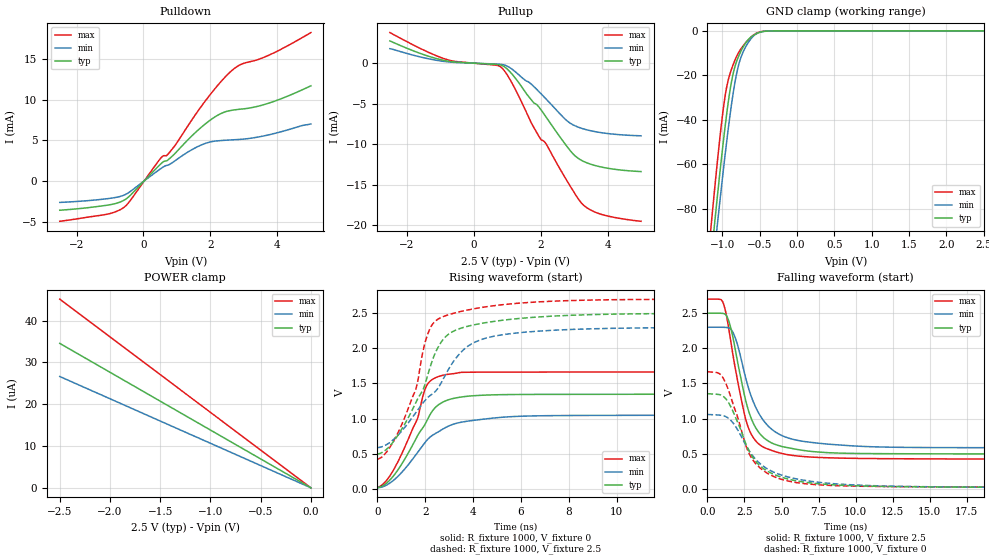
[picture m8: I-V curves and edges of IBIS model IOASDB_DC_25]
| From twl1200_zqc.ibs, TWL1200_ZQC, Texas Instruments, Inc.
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[Model]   IOASDB_DC_25
Model_type  I/O
Vinl=0.875
Vinh=1.625
Enable   Active-Low
Vref =   2.5
Rref =   1M
Cref =   15p
Vmeas =   1.25
| variable   typ   min   max
C_comp   3.71pF   3.05pF   4.62pF
| C_pullup   3.68pF   3.05pF   4.43pF
| C_pulldown   4.00pF   3.22pF   4.85pF
| C_tri-state   3.71pF   3.05pF   4.62pF
[Temperature Range]   40   100   -40
| Ambient temperature   25   85   -40
[Voltage range]   2.5   2.3   2.7
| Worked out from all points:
|   slope of the pulldown table from 0 to 0.375 V, typ, clamps not added: 235 ohm
|   slope of the pullup table from 0 to 0.375 V, typ, clamps not added: 4.33 kohm
|   GND clamp passes 1 mA (typ) near -0.53 V on its own axis
|   rising waveform, R_fixture 1000, V_fixture 0: 20-80 % time 1.37ns typ, 1.74ns min, 1.11ns max; typ from 0.018 V to 1.35 V
|   falling waveform, R_fixture 1000, V_fixture 2.5: 20-80 % time 1.42ns typ, 1.8ns min, 1.29ns max; typ from 2.5 V to 0.495 V
|   rising waveform, R_fixture 1000, V_fixture 2.5: 20-80 % time 1.59ns typ, 2.26ns min, 1.18ns max; typ from 0.495 V to 2.5 V
|   falling waveform, R_fixture 1000, V_fixture 0: 20-80 % time 2.05ns typ, 2.63ns min, 1.77ns max; typ from 1.35 V to 0.018 V
[GND Clamp]
| IOASDB_DC_25
|   Voltage   I(typ)   I(min)   I(max)
-2.5V     -598.9mA   -590.6mA   -610.7mA
-1.15V    -101.8mA   -113.6mA   -87.22mA
-1.105V   -86.79mA   -99.05mA   -71.51mA
-1.065V   -73.75mA   -86.36mA   -58.1mA
-1.005V   -55.04mA   -67.91mA   -39.7mA
-960mV    -42.05mA   -54.72mA   -28.6mA
-900mV    -27.23mA   -38.47mA   -19.48mA
-855mV    -19.12mA   -27.86mA   -15.13mA
-795mV    -12.45mA   -17.04mA   -10.54mA
-735mV    -8.086mA   -10.47mA   -7.334mA
-545mV    -1.273mA   -1.319mA   -1.079mA
2.5V      444.4pA    2.135uA    -3.613uA
[POWER Clamp]
| IOASDB_DC_25
|   Voltage   I(typ)   I(min)   I(max)
-2.5V     34.57uA    26.65uA    45.15uA
-90mV     1.246uA    964.2nA    1.63uA
-60mV     832.2nA    645.4nA    1.086uA
0V        0A         0A         0A
[Pulldown]
| IOASDB_DC_25
|   Voltage   I(typ)   I(min)   I(max)
-2.5V     -3.584mA   -2.621mA   -4.943mA
-1.07V    -2.952mA   -2.155mA   -4.055mA
-585mV    -2.357mA   -1.73mA    -3.231mA
510mV     2.093mA    1.517mA    2.803mA
695mV     2.5mA      1.936mA    3.157mA
925mV     3.328mA    2.454mA    4.301mA
1.545V    5.957mA    4.089mA    8.142mA
2.13V     7.887mA    4.918mA    11.35mA
2.575V    8.666mA    5.059mA    13.36mA
2.915V    8.858mA    5.143mA    14.36mA
3.66V     9.485mA    5.618mA    15.34mA
5V        11.72mA    7.033mA    18.27mA
[Pullup]
| IOASDB_DC_25
|   Voltage   I(typ)   I(min)   I(max)
-2.5V     2.747mA    1.789mA    3.778mA
-815mV    285.1uA    181uA      467.8uA
810mV     -231.5uA   -139.7uA   -468.2uA
1.14V     -1.314mA   -721.7uA   -2.411mA
1.75V     -4.664mA   -2.692mA   -7.583mA
1.95V     -5.412mA   -3.508mA   -9.026mA
2.165V    -6.66mA    -4.43mA    -9.972mA
2.78V     -10.24mA   -7.084mA   -14.47mA
3.005V    -11.35mA   -7.686mA   -15.98mA
3.23V     -12.02mA   -8.051mA   -17.31mA
3.8V      -12.81mA   -8.574mA   -18.65mA
5V        -13.39mA   -8.969mA   -19.52mA
[Ramp]
| IOASDB_DC_25
| variable   typ   min   max
dV/dt_r   0.80/1.37E-09   0.63/1.74E-09   0.99/1.11E-09
dV/dt_f   1.20/1.42E-09   1.03/1.80E-09   1.37/1.29E-09
R_load = 1000
[Rising Waveform]
| IOASDB_DC_25
R_fixture =   1000
C_fixture =   0
L_fixture =   0
V_fixture =   0
V_fixture_min = 0
V_fixture_max = 0
|   Time   V(typ)   V(min)   V(max)
0s        17.63mV    14.87mV    22.2mV
375ps     79.47mV    52.76mV    116.5mV
880ps     280.4mV    185.2mV    400.1mV
1.68ns    756.5mV    517.4mV    1.002V
2.12ns    1.003V     711.1mV    1.502V
2.645ns   1.217V     832.4mV    1.608V
3.595ns   1.312V     954.3mV    1.659V
7.055ns   1.345V     1.042V     1.663V
28.43ns   1.354V     1.056V     1.666V
239.9ns   1.355V     1.059V     1.667V
[Falling Waveform]
| IOASDB_DC_25
R_fixture =   1000
C_fixture =   0
L_fixture =   0
V_fixture =   2.5
V_fixture_min = 2.3
V_fixture_max = 2.7
|   Time   V(typ)   V(min)   V(max)
0s        2.5V       2.3V       2.7V
1.095ns   2.495V     2.299V     2.626V
1.435ns   2.391V     2.291V     2.286V
1.83ns    2.037V     2.175V     1.772V
2.56ns    1.276V     1.596V     1.01V
3.135ns   918.3mV    1.219V     716.7mV
3.81ns    726.7mV    965.4mV    591.3mV
4.655ns   627mV      800.9mV    525.2mV
7.43ns    525.2mV    652.2mV    448.7mV
239.9ns   494.9mV    586.9mV    420.8mV
[Rising Waveform]
| IOASDB_DC_25
R_fixture =   1000
C_fixture =   0
L_fixture =   0
V_fixture =   2.5
V_fixture_min = 2.3
V_fixture_max = 2.7
|   Time   V(typ)   V(min)   V(max)
0s        494.8mV    586.9mV    420.8mV
445ps     583.4mV    642.5mV    552mV
1.06ns    872.3mV    840.5mV    947.4mV
1.615ns   1.232V     1.088V     1.427V
2.06ns    1.565V     1.284V     2.157V
2.45ns    1.956V     1.397V     2.396V
3.015ns   2.211V     1.726V     2.482V
4.125ns   2.341V     2.096V     2.568V
8.18ns    2.471V     2.27V      2.681V
239.9ns   2.5V       2.3V       2.7V
[Falling Waveform]
| IOASDB_DC_25
R_fixture =   1000
C_fixture =   0
L_fixture =   0
V_fixture =   0
V_fixture_min = 0
V_fixture_max = 0
|   Time   V(typ)   V(min)   V(max)
0s        1.355V     1.059V     1.667V
725ps     1.344V     1.051V     1.649V
1.095ns   1.312V     1.04V      1.564V
1.785ns   1.074V     923mV      1.17V
2.705ns   584.2mV    581.3mV    555mV
3.58ns    322.7mV    355.3mV    293.6mV
5.41ns    142mV      172mV      113.8mV
8.78ns    55.24mV    70.39mV    46.02mV
29.37ns   21.1mV     19.34mV    25.24mV
239.9ns   17.93mV    15.21mV    22.51mV
